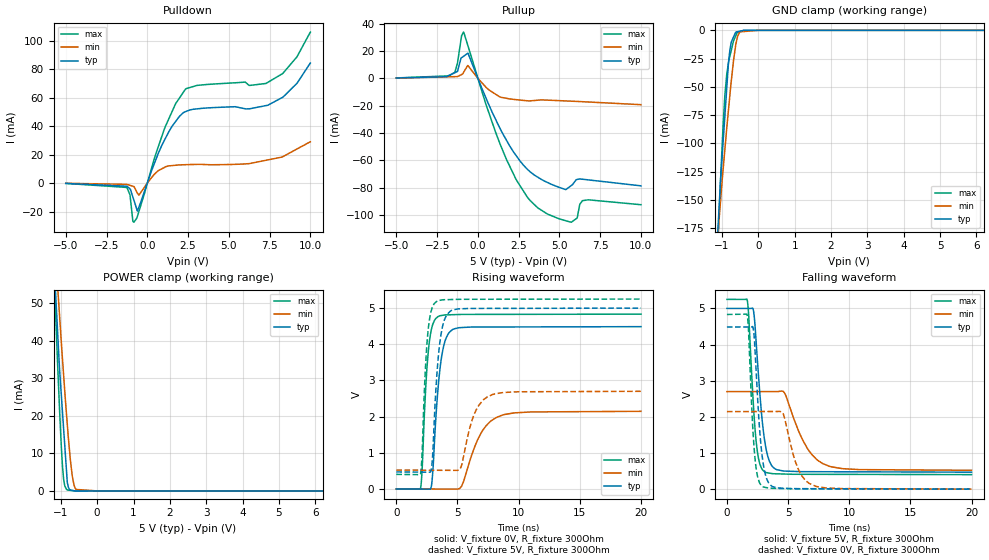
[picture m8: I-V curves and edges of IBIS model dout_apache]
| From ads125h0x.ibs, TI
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|   dout_apache Model
[Model]   dout_apache
Model_type   3-state
Polarity   Non-Inverting
Vmeas = 2.5
Vref = 0
Cref = 20pF
Rref = 100000
|   typ   min   max
C_comp   6.42217pF   5.72364pF   6.6322pF
|  Where Nom  PVT is Nominal Process,   5V,  27C
|   Fast PVT is Strong Process,   5.25V, -40C
|   Slow PVT is Weak Process,   2.7V, 135C
[Voltage Range]   5   2.7   5.25
|Junction Temperature
[Temperature Range]   27   135   -40
[Pullup Reference]   5   2.7   5.25
[Pulldown Reference]   0   0   -0
[Power Clamp Reference]   5   2.7   5.25
[GND Clamp Reference]   0   0   0
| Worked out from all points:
|   slope of the pulldown table from 0 to 0.75 V, typ, clamps not added: 32.8 ohm
|   slope of the pullup table from 0 to 0.75 V, typ, clamps not added: 35 ohm
|   GND clamp passes 1 mA (typ) near -0.55 V on its own axis
|   POWER clamp passes 1 mA (typ) near -0.79 V on its own axis
|   falling waveform, V_fixture 5V, R_fixture 300Ohm: 20-80 % time 685ps typ, 1.79ns min, 517ps max; typ from 5 V to 0.47 V
|   rising waveform, V_fixture 0V, R_fixture 300Ohm: 20-80 % time 616ps typ, 1.58ns min, 469ps max; typ from 0 V to 4.49 V
|   rising waveform, V_fixture 5V, R_fixture 300Ohm: 20-80 % time 541ps typ, 1.13ns min, 419ps max; typ from 0.47 V to 5 V
|   falling waveform, V_fixture 0V, R_fixture 300Ohm: 20-80 % time 550ps typ, 1.14ns min, 434ps max; typ from 4.49 V to 0 V
[Pulldown]
|   Voltage   I(typ)   I(min)   I(max)
-5V       -193.1uA   -112.3uA   -189.6uA
-1.25V    -2.138mA   -843.3uA   -3.017mA
-1.061V   -4.07mA    -1.537mA   -8.165mA
-883.6mV  -9.75mA    -2.187mA   -26.86mA
-821.5mV  -11.96mA   -2.414mA   -27.38mA
-607.1mV  -19.61mA   -7.003mA   -23.3mA
1.02V     29.38mA    10.84mA    37.11mA
2.336V    50.09mA    12.93mA    65.81mA
7.276V    54.36mA    16.03mA    69.89mA
8.308V    60.24mA    18.55mA    76.9mA
9.175V    69.97mA    23.93mA    88.52mA
10V       84.29mA    29.04mA    105.9mA
[GND Clamp]
|   Voltage   I(typ)   I(min)   I(max)
-5V       -2.828A    -2.084A    -3.614A
-1.128V   -186.1mA   -187.3mA   -202.1mA
-1.036V   -131.3mA   -149.9mA   -130.9mA
-969.2mV  -99.24mA   -123.5mA   -84.42mA
-917.5mV  -74.58mA   -104.6mA   -56.15mA
-867.4mV  -50.7mA    -86.21mA   -38.73mA
-821.4mV  -28.77mA   -70.6mA    -28.81mA
-782.3mV  -17.58mA   -57.42mA   -22.79mA
-607.1mV  -1.389mA   -10.44mA   -3.827mA
-507.3mV  -744.4uA   -1.362mA   -1.125mA
-131.8uV  -501.4pA   0A         0A
10V       0A         0A         0A
[Pullup]
|   Voltage   I(typ)   I(min)   I(max)
-5V       265.4uA    145.6uA    281.5uA
-1.412V   4.134mA    1.221mA    4.392mA
-997.9mV  15.12mA    2.749mA    31.18mA
-880.9mV  16.12mA    4.282mA    33.82mA
-607.1mV  18.45mA    9.263mA    23.7mA
1.382V    -37.18mA   -13.67mA   -48.68mA
3.195V    -68.25mA   -16.49mA   -89.26mA
5.178V    -80.54mA   -16.42mA   -103.4mA
5.731V    -78.41mA   -16.72mA   -105.2mA
6.089V    -73.97mA   -16.91mA   -102.2mA
6.408V    -73.78mA   -17.09mA   -89.51mA
10V       -78.63mA   -19.27mA   -92.43mA
[POWER Clamp]
|   Voltage   I(typ)   I(min)   I(max)
-5V       854.4mA    670.6mA    1.098A
-1.158V   55.64mA    64.8mA     50.98mA
-1.13V    50.2mA     60.7mA     44.16mA
-1.087V   42.17mA    54.4mA     33.68mA
-1.036V   32.55mA    46.85mA    21.96mA
-952.3mV  20.76mA    34.88mA    6.408mA
-890mV    11.96mA    26.41mA    1.31mA
-821.5mV  2.266mA    17.72mA    271.4uA
-736mV    264.2uA    8.179mA    144.7uA
-684.1mV  159uA      3.953mA    67.77uA
-580.5mV  2.729uA    395.7uA    1.632uA
10V       0A         0A         0A
[Ramp]
R_load = 300
|   typ   min   max
dV/dt_r   2.69207/6.16291e-10   1.28671/1.57306e-09   2.89953/4.68543e-10
dV/dt_f   2.71774/6.84608e-10   1.30632/1.79406e-09   2.90858/5.15995e-10
[Falling Waveform]
V_fixture = 5V
V_fixture_min = 2.7V
V_fixture_max = 5.25V
R_fixture = 300Ohm
C_fixture = 0F
|   Time   V(typ)   V(min)   V(max)
0s        5V         2.699V     5.25V
1.665ns   4.999V     2.699V     5.223V
2.141ns   4.987V     2.699V     2.471V
2.386ns   4.09V      2.699V     1.335V
3.057ns   1.407V     2.699V     486.9mV
4.004ns   549.9mV    2.699V     425.4mV
4.703ns   500.8mV    2.667V     418.4mV
6.745ns   483.9mV    1.044V     411.2mV
8.345ns   482.3mV    636.8mV    410.1mV
20ns      470.4mV    522.1mV    402.4mV
[Rising Waveform]
V_fixture = 0V
V_fixture_min = 0V
V_fixture_max = 0V
R_fixture = 300Ohm
C_fixture = 0F
|   Time   V(typ)   V(min)   V(max)
0s        149.8uV    1.394mV    15.49uV
1.98ns    -4.139mV   -796.6uV   18.03mV
2.624ns   -5.533mV   -1.509mV   3.835V
2.935ns   282.1mV    -1.853mV   4.502V
3.378ns   2.647V     -2.344mV   4.759V
3.872ns   3.954V     -2.89mV    4.807V
4.724ns   4.426V     -3.832mV   4.819V
6.945ns   4.477V     1.554V     4.826V
8.145ns   4.478V     1.97V      4.827V
20ns      4.487V     2.146V     4.833V
[Rising Waveform]
V_fixture = 5V
V_fixture_min = 2.7V
V_fixture_max = 5.25V
R_fixture = 300Ohm
C_fixture = 0F
|   Time   V(typ)   V(min)   V(max)
0s        470.4mV    522.1mV    402.4mV
1.98ns    465.6mV    518.6mV    420.5mV
2.586ns   464.1mV    517.5mV    4.343V
2.905ns   663.3mV    516.9mV    4.983V
3.29ns    3.041V     516.3mV    5.184V
3.812ns   4.54V      515.3mV    5.229V
4.624ns   4.95V      513.9mV    5.238V
6.563ns   4.991V     2.208V     5.244V
7.845ns   4.992V     2.608V     5.245V
20ns      5V         2.699V     5.25V
[Falling Waveform]
|Gnd
V_fixture = 0V
V_fixture_min = 0V
V_fixture_max = 0V
R_fixture = 300Ohm
C_fixture = 0F
|   Time   V(typ)   V(min)   V(max)
0s        4.487V     2.146V     4.833V
1.665ns   4.486V     2.147V     4.804V
2.261ns   4.062V     2.148V     980mV
2.639ns   1.814V     2.148V     204.6mV
2.884ns   906.7mV    2.148V     80.71mV
3.392ns   182.7mV    2.149V     31.8mV
4.515ns   27.53mV    2.13V      16.34mV
5.837ns   13.92mV    550.8mV    9.631mV
7.245ns   12.56mV    82.02mV    8.675mV
20ns      149.8uV    1.394mV    15.41uV
